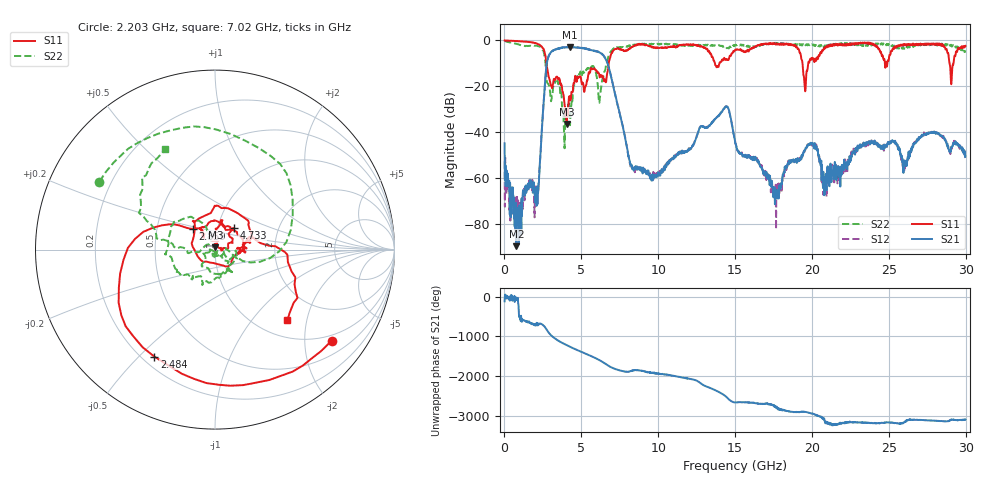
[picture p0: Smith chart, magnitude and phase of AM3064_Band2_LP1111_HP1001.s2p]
# Hz S DB R 50.0
!freq dBS11 angS11 dBS21 angS21 dBS12 angS12 dBS22 angS22
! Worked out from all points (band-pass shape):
!   1600 points, 10 MHz to 29.98 GHz, reference 50 ohm
!   highest |S21| = -2.81 dB at 4.246 GHz (marker M1); lowest = -89.6 dB at 778.5 MHz (marker M2)
!   |S21| within 3 dB of the highest: 2.954 GHz to 6.319 GHz (3.365 GHz wide, 72.6 % of centre)
!   lowest |S11| = -36.4 dB at 4.04 GHz (marker M3), VSWR 1.03, Z = 50.2 + j1.5 ohm
!   |S11| at or under -10 dB: 2.732 GHz to 6.784 GHz (4.052 GHz wide, 85.2 % of centre); 13.69 GHz to 13.98 GHz (286.7 MHz wide, 2.07 % of centre); 19.39 GHz to 19.76 GHz (369.8 MHz wide, 1.89 % of centre)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
!   |S22| runs from -47.0 to -0.1 dB; largest |S21 - S12| = 0.023
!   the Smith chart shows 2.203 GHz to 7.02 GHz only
!   S11 on the Smith chart (normalised r, x): 2.203 GHz: 0.84, -2.68; 2.484 GHz: 0.25, -0.56; 2.859 GHz: 0.76, +0.18; 4.733 GHz: 1.19, +0.29; 7.02 GHz: 1.33, -1.54
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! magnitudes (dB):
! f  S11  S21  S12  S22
! 10 MHz  0.0  -44.8  -52.8  -0.1
! 778.5 MHz  -0.3  -89.6  -69.6  -1.5
! 2.203 GHz  -1.7  -65.2  -65.9  -2.5
! 2.484 GHz  -3.3  -33.3  -33.4  -4.2
! 2.859 GHz  -15.4  -7.1  -7.1  -19.2
! 4.04 GHz  -36.4  -3.1  -3.0  -32.4
! 4.246 GHz  -24.3  -2.8  -2.9  -35.5
! 4.733 GHz  -16.0  -3.2  -3.1  -15.8
! 5.015 GHz  -18.3  -3.3  -3.2  -15.1
! 6.214 GHz  -15.8  -5.3  -5.3  -24.7
! 7.02 GHz  -5.0  -18.3  -18.1  -4.0
! 8.257 GHz  -2.9  -54.8  -54.6  -1.9
! 10 GHz  -3.3  -57.6  -57.2  -1.6
! 14.37 GHz  -8.5  -29.0  -29.0  -3.2
! 15 GHz  -4.1  -44.4  -44.0  -2.2
! 17.59 GHz  -1.3  -71.3  -69.8  -1.1
! 19.02 GHz  -2.9  -53.4  -52.5  -2.0
! 19.56 GHz  -22.2  -47.7  -47.7  -1.8
! 19.99 GHz  -7.6  -45.0  -44.7  -1.8
! 20.85 GHz  -3.4  -62.1  -64.9  -2.4
! 25 GHz  -8.6  -44.6  -44.8  -1.6
! 29.98 GHz  -2.4  -50.5  -51.2  -4.4
